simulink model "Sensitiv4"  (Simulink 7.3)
settings: Solver=ode45  StartTime=0.0  StopTime=10.0  RelTol=1e-3
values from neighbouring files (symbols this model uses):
  d2r = 1/r2d    (= 0.0174532925199)    [run.m]
  Kl3 = INFO.KFI(:,1:7)    [run.m]
  Kp3 = INFO.KFI(:,1:5)    [run.m]
  Thr = [470000, 470000, 470000, 0.245e7, 0.245e7]'    [run.m]
undefined symbols (not defined in the file or in its folder): Ap, Bp, Cp, Cyb, Cza, Dp, Mass, Qbar, Sref, TVC

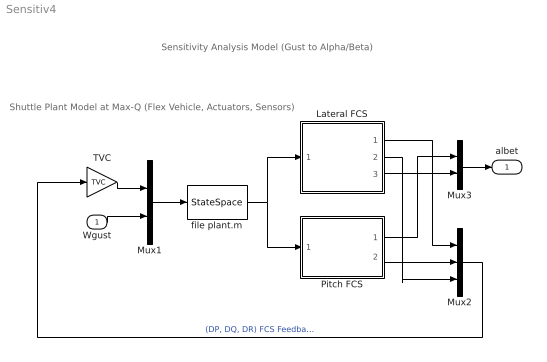
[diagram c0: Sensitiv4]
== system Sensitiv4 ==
  note: Shuttle Plant Model at Max-Q (Flex Vehicle, Actuators, Sensors)
  note: Sensitivity Analysis Model (Gust to Alpha/Beta)
  Wgust : Inport  OutDataType=sfix(16)  OutScaling=2^0
  Lateral FCS : Subsystem
  Mux1 : Mux  Inputs=[10,1]
  Mux2 : Mux  Inputs=3
  Mux3 : Mux  Inputs=2
  Pitch FCS : Subsystem
  TVC : Gain  Gain=TVC  Multiplication=Matrix(K*u)  ParameterDataType=sfix(16)  ParameterScaling=2^0  OutDataType=sfix(16)  OutScaling=2^0
  file plant.m : StateSpace  A=Ap  B=Bp  C=Cp  D=Dp
  albet : Outport
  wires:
  Mux1/1 -> file plant.m/1
  TVC/1 -> Mux1/1
  Wgust/1 -> Mux1/2
  Mux2/1 -> TVC/1  "(DP, DQ, DR) FCS Feedback"
  file plant.m/1 -> Lateral FCS/1(ym), Pitch FCS/1(ym)
  Lateral FCS/1(dP) -> Mux2/1
  Lateral FCS/2(dR) -> Mux2/3
  Pitch FCS/2(dQ) -> Mux2/2
  Pitch FCS/1(alf) -> Mux3/1
  Mux3/1 -> albet/1
  Lateral FCS/3(bet) -> Mux3/2

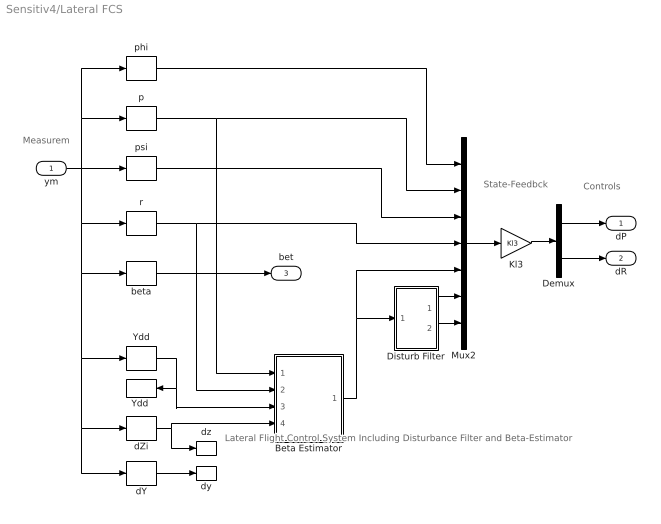
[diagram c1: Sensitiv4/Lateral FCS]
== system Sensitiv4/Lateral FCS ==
  note: Lateral Flight Control System Including Disturbance Filter and Beta-Estimator
  note: Measurem
  note: State-Feedbck
  note: Controls
  ym : Inport
  Beta Estimator : Subsystem
  Demux : Demux  Outputs=2
  Disturb Filter : Subsystem
  Kl3 : Gain  Gain=Kl3  Multiplication=Matrix(K*u)  ParameterDataType=sfix(16)  ParameterScaling=2^0  OutDataType=sfix(16)  OutScaling=2^0
  Mux2 : Mux  Inputs=7
  Ydd : Selector  InputPortWidth=30  IndexOptions=Index vector (dialog)  Indices=[7]  OutputSizes=1
  "Ydd " : ToWorkspace  VariableName=Ydd  SampleTime=-1  SaveFormat=Array
  beta : Selector  InputPortWidth=30  IndexOptions=Index vector (dialog)  Indices=[10]  OutputSizes=1
  dY : Selector  InputPortWidth=30  IndexOptions=Index vector (dialog)  Indices=[21:25]  OutputSizes=1
  dZi : Selector  InputPortWidth=30  IndexOptions=Index vector (dialog)  Indices=[26:30]  OutputSizes=1
  dy : ToWorkspace  VariableName=dy  SampleTime=-1  SaveFormat=Array
  dz : ToWorkspace  VariableName=dz  SampleTime=-1  SaveFormat=Array
  p : Selector  InputPortWidth=30  IndexOptions=Index vector (dialog)  Indices=[4]  OutputSizes=1
  phi : Selector  InputPortWidth=30  IndexOptions=Index vector (dialog)  Indices=[1]  OutputSizes=1
  psi : Selector  InputPortWidth=30  IndexOptions=Index vector (dialog)  Indices=[3]  OutputSizes=1
  r : Selector  InputPortWidth=30  IndexOptions=Index vector (dialog)  Indices=[6]  OutputSizes=1
  dP : Outport
  dR : Outport  Port=2
  bet : Outport  Port=3
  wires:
  Demux/1 -> dP/1
  Demux/2 -> dR/1
  Kl3/1 -> Demux/1
  dY/1 -> dy/1
  Beta Estimator/1(bethat) -> Disturb Filter/1(bet), Mux2/5
  dZi/1 -> dz/1, Beta Estimator/4(dz)
  Ydd/1 -> "Ydd "/1, Beta Estimator/3(Ydd)
  ym/1 -> r/1, beta/1, Ydd/1, dZi/1, dY/1, psi/1, phi/1, p/1
  r/1 -> Beta Estimator/2(r), Mux2/4
  psi/1 -> Mux2/3
  p/1 -> Beta Estimator/1(p), Mux2/2
  phi/1 -> Mux2/1
  Disturb Filter/2(x2) -> Mux2/7
  Disturb Filter/1(x1) -> Mux2/6
  Mux2/1 -> Kl3/1
  beta/1 -> bet/1

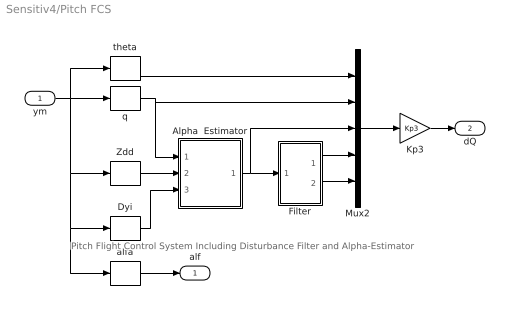
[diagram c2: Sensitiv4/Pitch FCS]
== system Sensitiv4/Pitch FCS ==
  note: Pitch Flight Control System Including Disturbance Filter and Alpha-Estimator
  ym : Inport
  Alpha  Estimator : Subsystem
  Dyi : Selector  InputPortWidth=30  IndexOptions=Index vector (dialog)  Indices=[21:25]  OutputSizes=1
  Filter : Subsystem
  Kp3 : Gain  Gain=Kp3  Multiplication=Matrix(K*u)  ParameterDataType=sfix(16)  ParameterScaling=2^0  OutDataType=sfix(16)  OutScaling=2^0
  Mux2 : Mux  Inputs=5
  Zdd : Selector  InputPortWidth=30  IndexOptions=Index vector (dialog)  Indices=[8]  OutputSizes=1
  alfa : Selector  InputPortWidth=30  IndexOptions=Index vector (dialog)  Indices=[9]  OutputSizes=1
  q : Selector  InputPortWidth=30  IndexOptions=Index vector (dialog)  Indices=[5]  OutputSizes=1
  theta : Selector  InputPortWidth=30  IndexOptions=Index vector (dialog)  Indices=[2]  OutputSizes=1
  alf : Outport
  dQ : Outport  Port=2
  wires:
  Mux2/1 -> Kp3/1
  Filter/1(x1) -> Mux2/4
  Filter/2(x2) -> Mux2/5
  theta/1 -> Mux2/1
  q/1 -> Mux2/2, Alpha  Estimator/1(q)
  ym/1 -> Dyi/1, alfa/1, Zdd/1, q/1, theta/1
  Alpha  Estimator/1(alphat) -> Filter/1(alfa), Mux2/3
  Zdd/1 -> Alpha  Estimator/2(Zdd)
  Dyi/1 -> Alpha  Estimator/3(delta)
  Kp3/1 -> dQ/1
  alfa/1 -> alf/1

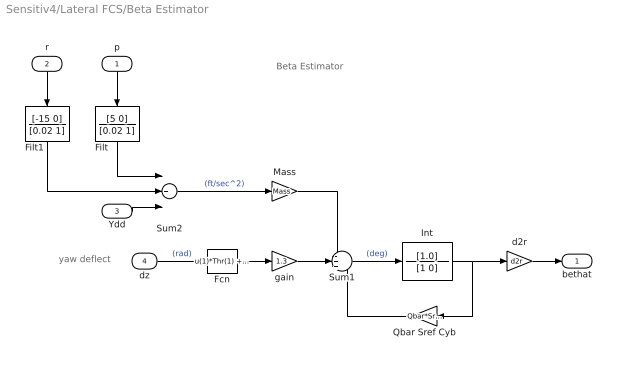
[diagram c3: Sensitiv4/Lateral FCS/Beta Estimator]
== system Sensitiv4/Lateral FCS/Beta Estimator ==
  note: yaw deflect
  note: Beta Estimator
  p : Inport
  r : Inport  Port=2
  Ydd : Inport  Port=3
  dz : Inport  Port=4  OutDataType=sfix(16)  OutScaling=2^0
  Fcn : Fcn  Expr=u(1)*Thr(1) +u(2)*Thr(2) +u(3)*Thr(3) +u(4)*Thr(4) +u(5)*Thr(5)
  Filt : TransferFcn  Numerator=[5 0]  Denominator=[0.02 1]
  Filt1 : TransferFcn  Numerator=[-15 0]  Denominator=[0.02 1]
  Int : TransferFcn  Numerator=[1.0]  Denominator=[1 0]
  Mass : Gain  Gain=Mass  ParameterDataType=sfix(16)  ParameterScaling=2^0  OutDataType=sfix(16)  OutScaling=2^0
  Qbar Sref Cyb : Gain  Gain=Qbar*Sref*Cyb  ParameterDataType=sfix(16)  ParameterScaling=2^0  OutDataType=sfix(16)  OutScaling=2^0
  Sum1 : Sum  Inputs=-++  OutDataType=sfix(16)  OutScaling=2^0
  Sum2 : Sum  Inputs=+++  OutDataType=sfix(16)  OutScaling=2^0
  d2r : Gain  Gain=d2r  ParameterDataType=sfix(16)  ParameterScaling=2^0  OutDataType=sfix(16)  OutScaling=2^0
  gain : Gain  Gain=1.3  ParameterDataType=sfix(16)  ParameterScaling=2^0  OutDataType=sfix(16)  OutScaling=2^0
  bethat : Outport  OutDataType=sfix(16)  OutScaling=2^0
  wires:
  Filt/1 -> Sum2/1
  p/1 -> Filt/1
  r/1 -> Filt1/1
  Ydd/1 -> Sum2/3
  gain/1 -> Sum1/2
  Fcn/1 -> gain/1
  Int/1 -> Qbar Sref Cyb/1, d2r/1
  d2r/1 -> bethat/1
  Mass/1 -> Sum1/1
  Sum2/1 -> Mass/1  "(ft/sec^2)"
  dz/1 -> Fcn/1  "(rad)"
  Qbar Sref Cyb/1 -> Sum1/3
  Sum1/1 -> Int/1  "(deg)"
  Filt1/1 -> Sum2/2

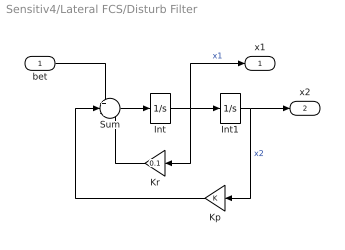
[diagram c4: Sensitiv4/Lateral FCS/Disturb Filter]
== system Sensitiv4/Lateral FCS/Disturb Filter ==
  bet : Inport  OutDataType=sfix(16)  OutScaling=2^0
  Int : Integrator
  Int1 : Integrator
  Kp : Gain  ParameterDataType=sfix(16)  ParameterScaling=2^0  OutDataType=sfix(16)  OutScaling=2^0
  Kr : Gain  Gain=0.1  ParameterDataType=sfix(16)  ParameterScaling=2^0  OutDataType=sfix(16)  OutScaling=2^0
  Sum : Sum  Inputs=+--  OutDataType=sfix(16)  OutScaling=2^0
  x1 : Outport  OutDataType=sfix(16)  OutScaling=2^0
  x2 : Outport  Port=2  OutDataType=sfix(16)  OutScaling=2^0
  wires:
  bet/1 -> Sum/1
  Kp/1 -> Sum/2
  Kr/1 -> Sum/3
  Int1/1 -> x2/1, Kp/1  "x2"
  Sum/1 -> Int/1
  Int/1 -> x1/1, Kr/1, Int1/1  "x1"

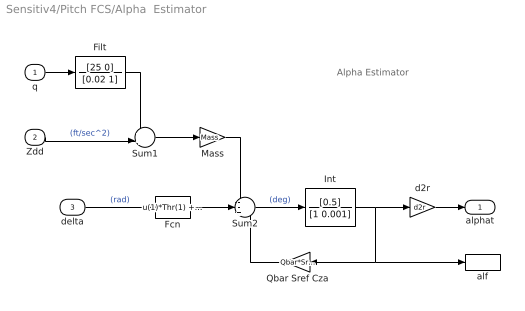
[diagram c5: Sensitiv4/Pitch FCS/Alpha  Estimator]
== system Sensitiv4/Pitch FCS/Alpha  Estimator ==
  note: Alpha Estimator
  q : Inport  OutDataType=sfix(16)  OutScaling=2^0
  Zdd : Inport  Port=2  OutDataType=sfix(16)  OutScaling=2^0
  delta : Inport  Port=3  OutDataType=sfix(16)  OutScaling=2^0
  Fcn : Fcn  Expr=u(1)*Thr(1) +u(2)*Thr(2) +u(3)*Thr(3) +u(4)*Thr(4) +u(5)*Thr(5)
  Filt : TransferFcn  Numerator=[25 0]  Denominator=[0.02 1]
  Int : TransferFcn  Numerator=[0.5]  Denominator=[1 0.001]
  Mass : Gain  Gain=Mass  ParameterDataType=sfix(16)  ParameterScaling=2^0  OutDataType=sfix(16)  OutScaling=2^0
  Qbar Sref Cza : Gain  Gain=Qbar*Sref*Cza  ParameterDataType=sfix(16)  ParameterScaling=2^0  OutDataType=sfix(16)  OutScaling=2^0
  Sum1 : Sum  Inputs=++|  OutDataType=sfix(16)  OutScaling=2^0
  Sum2 : Sum  Inputs=--+  OutDataType=sfix(16)  OutScaling=2^0
  alf : ToWorkspace  VariableName=alphat  SampleTime=-1  SaveFormat=Array
  d2r : Gain  Gain=d2r  ParameterDataType=sfix(16)  ParameterScaling=2^0  OutDataType=sfix(16)  OutScaling=2^0
  alphat : Outport  OutDataType=sfix(16)  OutScaling=2^0
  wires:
  Int/1 -> alf/1, Qbar Sref Cza/1, d2r/1
  d2r/1 -> alphat/1
  Mass/1 -> Sum2/1
  delta/1 -> Fcn/1  "(rad)"
  Qbar Sref Cza/1 -> Sum2/3
  Sum2/1 -> Int/1  "(deg)"
  q/1 -> Filt/1
  Zdd/1 -> Sum1/2  "(ft/sec^2)"
  Sum1/1 -> Mass/1
  Filt/1 -> Sum1/1
  Fcn/1 -> Sum2/2

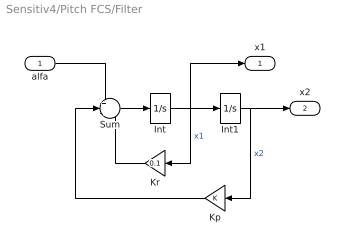
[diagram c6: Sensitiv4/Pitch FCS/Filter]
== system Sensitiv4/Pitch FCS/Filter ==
  alfa : Inport  OutDataType=sfix(16)  OutScaling=2^0
  Int : Integrator
  Int1 : Integrator
  Kp : Gain  ParameterDataType=sfix(16)  ParameterScaling=2^0  OutDataType=sfix(16)  OutScaling=2^0
  Kr : Gain  Gain=0.1  ParameterDataType=sfix(16)  ParameterScaling=2^0  OutDataType=sfix(16)  OutScaling=2^0
  Sum : Sum  Inputs=+--  OutDataType=sfix(16)  OutScaling=2^0
  x1 : Outport  OutDataType=sfix(16)  OutScaling=2^0
  x2 : Outport  Port=2  OutDataType=sfix(16)  OutScaling=2^0
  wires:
  Int/1 -> Int1/1, Kr/1, x1/1  "x1"
  Sum/1 -> Int/1
  Int1/1 -> Kp/1, x2/1  "x2"
  Kr/1 -> Sum/3
  Kp/1 -> Sum/2
  alfa/1 -> Sum/1
